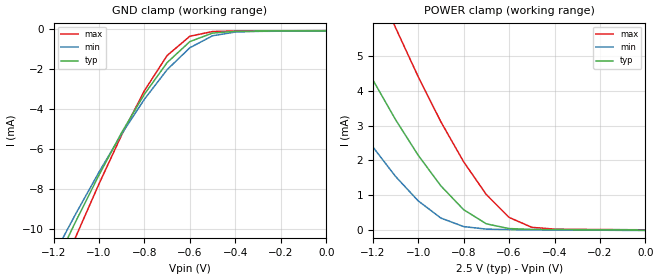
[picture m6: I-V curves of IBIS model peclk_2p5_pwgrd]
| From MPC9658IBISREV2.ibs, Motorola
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|This model is for a 2.5V Pecl Input with a 25,000 ohm pull_down
[Model]   peclk_2p5_pwgrd
Model_type   Input
Vmeas=1.25
Vinl=0.7
Vinh=1.7
| Variable   typ   min   max
C_comp   5p   5p   5p
[Temperature Range]   27.00   100.00   -45.00
[Power Clamp Reference]   2.50V   2.25V   2.75V
[Gnd Clamp Reference]   0.000V   0.000V   0.000V
[Voltage Range]   2.50V   2.25V   2.75V
[Pulldown Reference]   0.000V   0.000V   0.000V
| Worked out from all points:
|   GND clamp passes 1 mA (typ) near -0.63 V on its own axis
|   POWER clamp passes 1 mA (typ) near -0.86 V on its own axis
[GND_clamp]
| voltage   I(typ)   I(min)   I(max)
-2.5V     -45.01mA   -42.15mA   -48.72mA
-1.2V     -11.92mA   -11.32mA   -12.99mA
-1.1V     -9.563mA   -9.191mA   -10.33mA
-1V       -7.298mA   -7.155mA   -7.742mA
-900mV    -5.174mA   -5.246mA   -5.294mA
-800mV    -3.26mA    -3.513mA   -3.086mA
-700mV    -1.682mA   -2.036mA   -1.33mA
-600mV    -635.3uA   -942.6uA   -367.1uA
-500mV    -210uA     -344uA     -133.5uA
-400mV    -124uA     -158.5uA   -106.1uA
1.08fV    -99.01uA   -108.9uA   -89.1uA
[POWER_clamp]
| voltage   I(typ)  I(min)  I(max)
-2.5V     23.81mA    19.16mA    29.58mA
-1.6V     9.684mA    6.706mA    13.85mA
-1.5V     8.252mA    5.519mA    12.16mA
-1.3V     5.557mA    3.352mA    8.885mA
-1.1V     3.177mA    1.545mA    5.818mA
-1V       2.15mA     841.2uA    4.407mA
-900mV    1.27mA     346.2uA    3.11mA
-800mV    587.9uA    102.4uA    1.963mA
-700mV    181.2uA    28.88uA    1.02mA
-600mV    45.26uA    15.08uA    365.9uA
-500mV    21.73uA    10.02uA    80.89uA
1.08fV    72.56pA    -9.897uA   9.901uA
